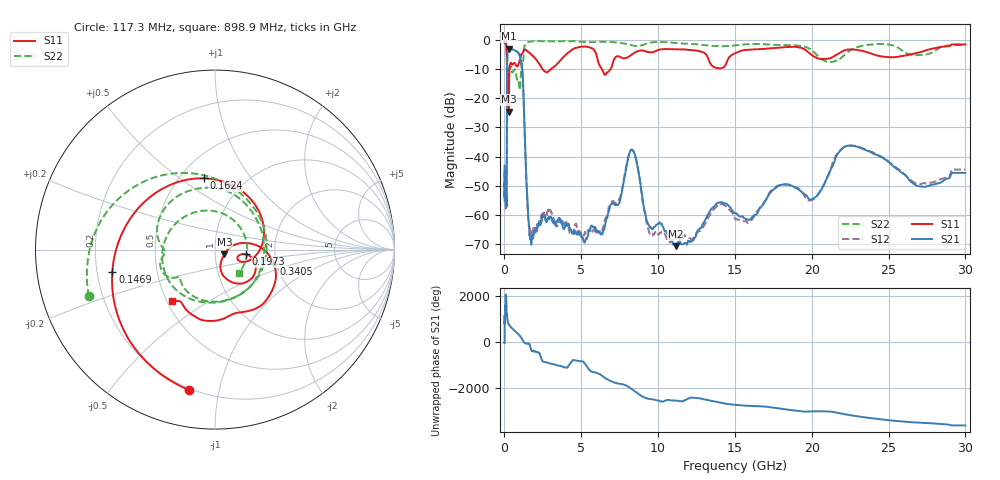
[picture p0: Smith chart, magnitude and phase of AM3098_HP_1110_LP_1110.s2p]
! Date/Time: Thu, Feb 28, 2019 8:47 AM
! Network Analyzer: Agilent Technologies E8364B Rev: A.07.50.67
! Sweep from 0.010 to 30.000 GHz, 1601 Points, Sweep Type: LOG
! Power Supply: 5.022 V, 0.002 A
# Hz S DB R 50
!freq MagS11 AngS11 MagS21 AngS21 MagS12 AngS12 MagS22 AngS22
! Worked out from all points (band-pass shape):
!   1601 points, 10 MHz to 30 GHz, reference 50 ohm
!   highest |S21| = -3.14 dB at 296 MHz (marker M1); lowest = -70.6 dB at 11.14 GHz (marker M2)
!   |S21| within 3 dB of the highest: 183.7 MHz to 1.028 GHz (844.8 MHz wide, 139 % of centre)
!   lowest |S11| = -24.6 dB at 266.5 MHz (marker M3), VSWR 1.13, Z = 55.5 - j2.95 ohm
!   |S11| at or under -10 dB: 169.7 MHz to 332.3 MHz (162.6 MHz wide, 64.8 % of centre); 2.471 GHz to 3.033 GHz (562.3 MHz wide, 20.4 % of centre); 6.329 GHz to 6.917 GHz (587.7 MHz wide, 8.87 % of centre)
!   |S22| runs from -17.2 to -0.5 dB; largest |S21 - S12| = 0.011
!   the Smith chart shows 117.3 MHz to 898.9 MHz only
!   S11 on the Smith chart (normalised r, x): 117.3 MHz: 0.19, -0.81; 146.9 MHz: 0.26, -0.10; 162.4 MHz: 0.65, +0.62; 197.3 MHz: 1.42, -0.08; 340.5 MHz: 1.93, -0.34; 898.9 MHz: 0.54, -0.35
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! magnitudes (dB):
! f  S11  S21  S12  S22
! 10 MHz  -0.4  -43.1  -47.1  -0.6
! 38.04 MHz  -0.3  -52.2  -50.6  -0.8
! 117.3 MHz  -2.0  -53.6  -53.7  -2.5
! 144.7 MHz  -4.3  -51.9  -48.6  -5.4
! 146.9 MHz  -4.7  -49.1  -46.5  -6.0
! 162.4 MHz  -7.9  -22.3  -22.2  -10.8
! 197.3 MHz  -15.1  -4.6  -4.6  -11.4
! 266.5 MHz  -24.6  -3.2  -3.2  -11.2
! 296 MHz  -15.1  -3.1  -3.1  -10.5
! 340.5 MHz  -9.5  -3.3  -3.2  -9.1
! 550.5 MHz  -8.4  -3.4  -3.4  -11.1
! 898.9 MHz  -8.6  -4.5  -4.5  -14.7
! 1.178 GHz  -4.7  -11.3  -11.2  -8.7
! 1.68 GHz  -4.8  -68.0  -65.5  -0.7
! 2.084 GHz  -6.9  -65.6  -65.0  -0.5
! 6.141 GHz  -8.2  -65.6  -65.7  -0.8
! 7.926 GHz  -6.2  -43.9  -43.3  -1.5
! 8.416 GHz  -4.6  -38.4  -38.4  -2.1
! 11.14 GHz  -3.3  -70.6  -67.9  -1.1
! 20.1 GHz  -5.6  -54.4  -54.6  -4.1
! 22.56 GHz  -3.4  -36.3  -36.2  -3.5
! 30 GHz  -1.6  -45.6  -44.4  -1.9
